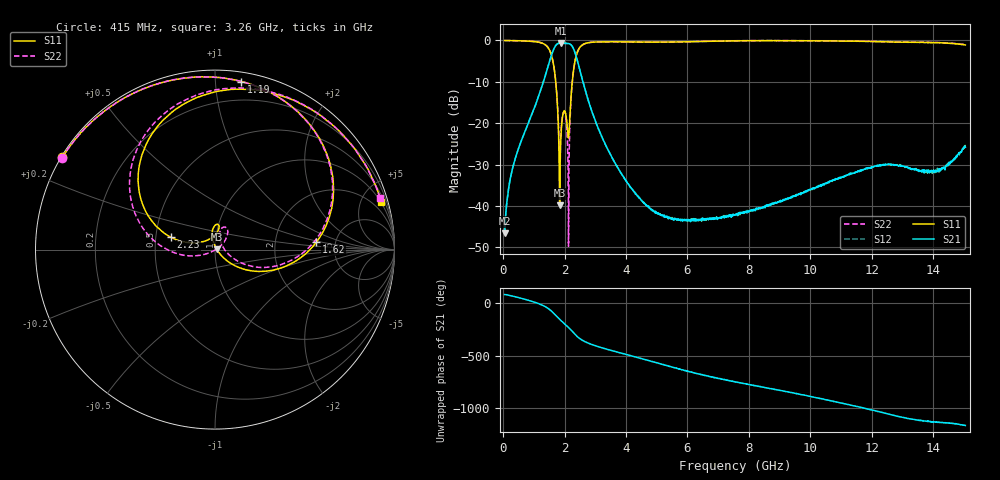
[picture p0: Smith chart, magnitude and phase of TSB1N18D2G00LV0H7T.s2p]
! TSB1N18D2G00LV0H7T  S-PARAMETER MODEL  ( General Type )
! Model Generated by TAIYO YUDEN Corporation (https://www.yuden.co.jp/en/)
! Version 1.0
! TAIYO YUDEN Control No. 20190830
! Copyright(c) 2019 TAIYO YUDEN CO.,LTD. All Rights Reserved.
! Products Name : Multilayer Ceramic Devices
! Characteristics :
!  Passband freq : 1805-2200MHz ( At Passband , Insertion Loss : 1.8dB , VSWR 2.0 ),
!  Attenuation : 16dBmin at 600 to 735MHz, 22dBmin at 3610 to 6600MHz , Impedance : 50 Ohm ,
!  Case Size : 1.6 x 0.8 / 0.063 x 0.031 [mm/inch] , Thickness : 0.65 / 0.026 [mm/inch]
!  (Conditions: Temperature = 25 degC , DC Bias Current/Voltage = 0A / 0V)
! External Node Assignments :
!  1  o---|-------|---o  2
!  |  BPF  |
! GND o---|-------|---o GND
! Frequency Range : 50MHz  -  15.05GHz  [ 1901 STEP ]
# MHZ S RI R 50
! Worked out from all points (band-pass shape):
!   1901 points, 50 MHz to 15.05 GHz, reference 50 ohm
!   highest |S21| = -0.63 dB at 1.87 GHz (marker M1); lowest = -46.6 dB at 50 MHz (marker M2)
!   |S21| within 3 dB of the highest: 1.572 GHz to 2.371 GHz (799.3 MHz wide, 40.5 % of centre)
!   lowest |S11| = -39.8 dB at 1.84 GHz (marker M3), VSWR 1.02, Z = 51 + j0.159 ohm
!   |S11| at or under -10 dB: 1.714 GHz to 2.252 GHz (537.7 MHz wide, 27.1 % of centre)
!   |S22| runs from -49.8 to 0.0 dB; largest |S21 - S12| = 0.0029
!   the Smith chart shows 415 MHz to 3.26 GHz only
!   S11 on the Smith chart (normalised r, x): 415 MHz: 0.00, +0.28; 1.19 GHz: 0.06, +1.17; 1.62 GHz: 3.55, +0.43; 2.23 GHz: 0.60, +0.09; 3.26 GHz: 0.93, +6.95
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50  -0.9959 0.068  0.000917 0.00456  0.000874 0.00463  -0.9951 0.0681
415  -0.851 0.5144  0.0217 0.0328  0.0216 0.0329  -0.8514 0.5126
1190  0.1465 0.9362  0.2246 -0.0431  0.2252 -0.044  0.1418 0.9376
1620  0.5645 0.0408  -0.000473 -0.7394  -0.000665 -0.739  0.5662 0.0613
1840  0.0101 0.00156  -0.8453 -0.3848  -0.8455 -0.3849  0.0435 0.0161
1870  -0.0106 0.0472  -0.8932 -0.2587  -0.893 -0.2592  0.0276 0.0567
2010  0.0186 0.139  -0.8642 0.3213  -0.8639 0.3207  0.0675 0.1151
2130  -0.0334 0.0576  -0.5533 0.7337  -0.5535 0.7327  0.0031 -0.000991
2230  -0.2457 0.0691  -0.0935 0.8667  -0.0945 0.8657  -0.2446 -0.0107
2550  -0.0556 0.8625  0.3646 0.0665  0.3635 0.0672  -0.1155 0.8561
3260  0.9256 0.2673  0.0217 -0.0592  0.0215 -0.059  0.9187 0.2884
4260  0.4386 -0.854  -0.0128 -0.00759  -0.0127 -0.0076  0.4289 -0.856
5050  -0.5423 -0.7864  -0.00697 0.0043  -0.00678 0.00426  -0.5691 -0.7661
6050  -0.9097 0.3258  0.00244 0.0062  0.00256 0.00617  -0.8912 0.3753
6790  -0.3355 0.9194  0.00684 0.0019  0.00676 0.00218  -0.2862 0.9374
7550  0.4452 0.8834  0.00684 -0.00385  0.00692 -0.00381  0.4839 0.8666
8750  0.9938 -0.082  -0.000953 -0.0106  -0.00113 -0.0104  0.9947 -0.0923
10050  0.2442 -0.96  -0.0157 -0.00254  -0.0159 -0.00242  0.2857 -0.9533
11440  -0.8415 -0.5011  -0.00488 0.0247  -0.00496 0.0245  -0.7941 -0.5826
12550  -0.8693 0.4089  0.0292 0.0133  0.0288 0.0127  -0.9236 0.2959
13920  0.0348 0.9395  0.0169 -0.0199  0.0179 -0.0201  -0.1214 0.9376
15050  0.8398 0.2688  0.00556 -0.051  0.00547 -0.052  0.7695 0.4453
